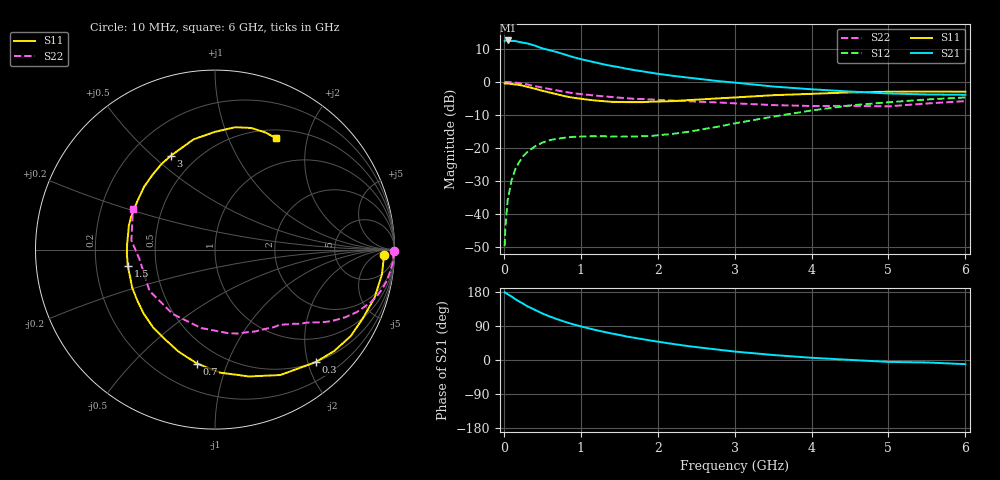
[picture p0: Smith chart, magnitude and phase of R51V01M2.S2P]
! SIEMENS Small Signal Semiconductors
! BFR183
! Si NPN RF Bipolar Junction Transistor in SOT23
! VCE = 1 V  IC = 1.2 mA
! Common Emitter S-Parameters:  May  1996
# GHz  S  MA  R  50
!  f  S11  S21  S12  S22
! GHz  MAG  ANG  MAG  ANG  MAG  ANG  MAG  ANG
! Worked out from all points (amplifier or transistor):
!   36 points, 10 MHz to 6 GHz, reference 50 ohm
!   highest |S21| = 12.6 dB at 50 MHz (marker M1)
!   |S21| within 3 dB of that: start of sweep to 602.5 MHz
!   unconditionally stable (mu >= 1): 1.557 GHz to 3.186 GHz
!   at 250 MHz: K = 0.17, MSG = 17.2 dB, |S12| = -22.6 dB
!   at 1.4 GHz: K = 0.92, MSG = 10.7 dB, |S12| = -16.6 dB
!   at 6 GHz: K = 0.97, MSG = 0.4 dB, |S12| = -4.8 dB
!   S11 on the Smith chart (normalised r, x): 10 MHz: 27, -14; 300 MHz: 0.50, -2.14; 700 MHz: 0.36, -0.79; 1.5 GHz: 0.34, -0.08; 3 GHz: 0.36, +0.57; 6 GHz: 0.61, +1.52
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0.01  0.9441 -1.7  4.144 179.1  0.0032 87.2  0.998 -0.6
0.02  0.9414 -3.2  4.235 177.4  0.0061 87.2  0.9926 -1.4
0.05  0.94 -8.5  4.243 173.7  0.016 84.7  0.9952 -3.5
0.1  0.9288 -16.7  4.157 167.5  0.0319 80.1  0.9846 -6.9
0.15  0.9086 -24.9  4.161 160.3  0.0472 75.0  0.9727 -10.3
0.3  0.841 -48.2  3.841 142.4  0.085 62.5  0.9132 -19.0
0.4  0.7879 -62.5  3.553 132.7  0.1041 54.8  0.8622 -23.9
0.5  0.7317 -75.0  3.219 122.9  0.1193 48.8  0.8169 -27.5
0.6  0.6856 -87.8  3.009 114.7  0.1304 43.9  0.7758 -30.5
0.7  0.6425 -99.0  2.805 107.2  0.137 39.7  0.7364 -33.2
0.8  0.6035 -109.7  2.577 100.4  0.1422 36.3  0.7004 -35.4
0.9  0.573 -118.8  2.373 94.3  0.1459 33.8  0.6722 -37.1
1.1  0.5339 -138.1  2.079 83.7  0.1489 30.2  0.6334 -40.5
1.3  0.508 -155.2  1.839 74.3  0.1492 28.9  0.6011 -43.4
1.5  0.4943 -169.5  1.666 66.2  0.147 30.0  0.574 -46.5
1.9  0.4984 164.3  1.384 51.6  0.1503 35.4  0.5402 -53.3
2.2  0.5095 148.4  1.232 42.3  0.1623 41.1  0.5189 -59.1
3  0.5782 115.2  0.974 22.3  0.2337 48.9  0.4713 -81.1
3.5  0.6261 100.9  0.848 13.2  0.2965 46.6  0.4436 -100.1
4.5  0.6912 80.6  0.712 0.3  0.438 33.9  0.4314 -147.8
5.5  0.7106 66.5  0.643 -6.5  0.5394 18.3  0.4686 173.8
6  0.7071 61.1  0.635 -11.0  0.5787 8.9  0.5092 153.9
